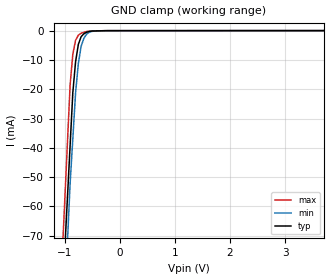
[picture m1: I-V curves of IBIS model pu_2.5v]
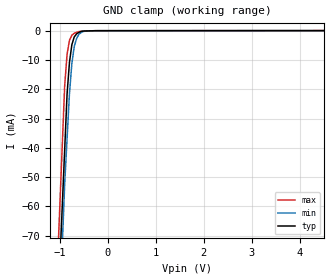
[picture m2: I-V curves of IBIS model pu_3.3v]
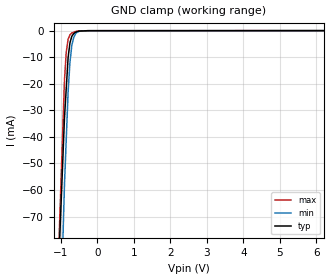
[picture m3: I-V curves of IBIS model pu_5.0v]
| Teraspeed Modeling Services.
| http://www.teraspeed.com
[IBIS Ver]   4.0
[Comment Char] |_char
[File Name]   pca9617dp.ibs
[File Rev]   3.0
[Source]  Measured and created by Teraspeed Consulting Group LLC
[Date]   10-19-2012
[Notes]   Quality Check of this IBIS model: Model Passes IBIS Check
   Model parses into ICX IS. Simulation done with Hyperlynx.
   1. MIN TYP MAX information is based on Temperature and Voltage
   characteristics only.
   2. Package data measured using Tektronix IConnect Software.
[Disclaimer]
| Use: Teraspeed Consulting Group LLC ("Teraspeed") has
| licensed IBIS models to specific integrated circuit
| suppliers ("IC Vendors") for use and distribution as
| follows: Each IC Vendor may use IBIS Models, and distribute
| them to IC Vendor's customers to use solely for developing
| printed circuit board designs. Users of this model may
| modify the IBIS model to suit its specific applications but
| rights to derivative works and such modifications shall belong
| to Teraspeed. No other distribution of these materials is
| permitted.
| DISCLAIMER OF WARRANTY: UNLESS OTHERWISE AGREED TO IN WRITING
| TERASPEED DISCLAIMS AND USER WAIVES ALL WARRANTIES, EXPRESS
| OR IMPLIED, INCLUDING WARRANTIES OF MERCHANTABILITY AND
| FITNESS FOR A PARTICULAR PURPOSE. IN NO EVENT SHALL
| TERASPEED BE LIABLE FOR ANY DIRECT OR INDIRECT DAMAGES,
| WHETHER IN CONTRACT OR TORT, INCLUDING, WITHOUT LIMITATION,
| LOST PROFITS, BUSINESS INTERRUPTION, OR LOST INFORMATION
| ARISING OUT OF THE USE OF OR THE INABILITY TO USE THE MODEL,
| EVEN IF TERASPEED HAS BEEN ADVISED OF THE POSSIBILITY OF SUCH
| DAMAGES.
[Copyright]
| This file is the legal property of Teraspeed Copyright(c) 2012.
| All other rights are reserved.
[Component] PCA9617DP
[Manufacturer] NXP Semiconductors
| TSSOP08/SOT505-1
[Package]
| variable   typ   min   max
R_pkg  1.100E-02  1.000E-02  1.200E-01
L_pkg  2.140E-09  2.040E-09  2.240E-09
C_pkg  5.910E-13  5.470E-13  6.350E-13
[Pin] signal_name  model_name  R_pin  L_pin C_pin
1  VCCA  POWER   1.200E-02 2.240E-09 5.470E-13
2  SCLA  io_side_a 1.000E-02 2.040E-09 6.350E-13
3  SDAA  io_side_a 1.000E-02 2.040E-09 6.350E-13
4  GND   GND   1.200E-02 2.240E-09 5.470E-13
5  EN   in_pu   1.200E-02 2.240E-09 5.470E-13
6  SDAB  io_side_b 1.000E-02 2.040E-09 6.350E-13
7  SCLB  io_side_b 1.000E-02 2.040E-09 6.350E-13
8  VCCB  POWER   1.200E-02 2.240E-09 5.470E-13
[Model selector] in_pu
pu_2.5v   input pin w/int pu,vccb=2.5v
pu_3.3v   input pin w/int pu,vccb=3.3v
pu_5.0v   input pin w/int pu,vccb=5.0v
[Model selector] io_side_b
sdab_2.5v  open drain io,vccb=2.5v
sdab_3.3v  open drain io,vccb=3.3v
sdab_5.0v  open drain io,vccb=5.0v
[Model selector] io_side_a
scla_0.95v  open drain io,vcca=0.95v
scla_1.8v   open drain io,vcca=1.8v
scla_2.5v   open drain io,vcca=2.5v
scla_3.3v   open drain io,vcca=3.3v
scla_5.0v   open drain io,vcca=5.0v
| Models and submodels in the file (11): pu_2.5v (Input), pu_3.3v (Input), pu_5.0v (Input), scla_0.95v (Open_drain), scla_1.8v (Open_drain), scla_2.5v (Open_drain), scla_3.3v (Open_drain), scla_5.0v (Open_drain), sdab_2.5v (Open_drain), sdab_3.3v (Open_drain), sdab_5.0v (Open_drain)
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[Model] pu_2.5v
Model_type Input
Vinl = 750.000mV
Vinh = 1.75000V
C_comp 600.000fF 595.000fF 605.000fF
| variable typ   min   max
[Voltage Range] 2.50000V 2.25000V 2.75000V
[POWER Clamp Reference] 2.50000V 2.25000V 2.75000V
[GND Clamp Reference] 0.00000V 0.00000V 0.00000V
[Temperature Range]   25   85   -40
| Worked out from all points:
|   GND clamp passes 1 mA (typ) near -0.64 V on its own axis
[GND Clamp]
-2.5V     -627.1mA   -717.8mA   -670.4mA
-900mV    -39.48mA   -52.45mA   -18.76mA
-850mV    -21.11mA   -36.83mA   -7.99mA
-800mV    -10.6mA    -21.21mA   -3.277mA
-750mV    -4.707mA   -11.24mA   -1.562mA
-700mV    -2.099mA   -5.37mA    -892uA
-650mV    -1.081mA   -2.621mA   -599.1uA
-600mV    -559.7uA   -1.191mA   -306.3uA
-550mV    -288.3uA   -553.5uA   -144.6uA
-450mV    -112.8uA   -112.5uA   -100.7uA
5V        11.01uA    12.15uA    11.05uA
[POWER Clamp]
-2.5V     0A         0A         0A
5V        0A         0A         0A
[Model] pu_3.3v
Model_type Input
Vinl = 990.000mV
Vinh = 2.31000V
C_comp 600.000fF 595.000fF 605.000fF
| variable typ   min   max
[Voltage Range] 3.30000V 2.97000V 3.63000V
[POWER Clamp Reference] 3.30000V 2.97000V 3.63000V
[GND Clamp Reference] 0.00000V 0.00000V 0.00000V
[Temperature Range]   25   85   -40
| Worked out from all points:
|   GND clamp passes 1 mA (typ) near -0.64 V on its own axis
[GND Clamp]
-3.3V     -958.1mA   -1.054A    -992.5mA
-900mV    -40.76mA   -52.47mA   -18.88mA
-850mV    -21.65mA   -36.93mA   -8.066mA
-800mV    -10.81mA   -21.4mA    -3.309mA
-750mV    -4.779mA   -11.22mA   -1.574mA
-700mV    -2.121mA   -5.352mA   -898.2uA
-650mV    -1.09mA    -2.612mA   -604.4uA
-600mV    -564.5uA   -1.187mA   -310.5uA
-550mV    -291.8uA   -553.5uA   -148.8uA
-450mV    -115.7uA   -113.5uA   -104.6uA
6.6V      16.4uA     15.45uA    14uA
[POWER Clamp]
-3.3V     0A         0A         0A
6.6V      0A         0A         0A
[Model] pu_5.0v
Model_type Input
Vinl = 1.50000V
Vinh = 3.50000V
C_comp 600.000fF 595.000fF 605.000fF
| variable typ   min   max
[Voltage Range] 5.00000V 4.50000V 5.50000V
[POWER Clamp Reference] 5.00000V 4.50000V 5.50000V
[GND Clamp Reference] 0.00000V 0.00000V 0.00000V
[Temperature Range]   25   85   -40
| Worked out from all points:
|   GND clamp passes 1 mA (typ) near -0.64 V on its own axis
[GND Clamp]
-5V       -1.459A    -2.026A    -1.674A
-900mV    -32.74mA   -57.89mA   -18.48mA
-850mV    -21.38mA   -40.39mA   -7.863mA
-800mV    -10.01mA   -22.89mA   -3.237mA
-750mV    -4.6mA     -11.87mA   -1.553mA
-700mV    -2.151mA   -5.589mA   -892.8uA
-650mV    -1.158mA   -2.704mA   -602.4uA
-600mV    -624.7uA   -1.224mA   -312uA
-500mV    -158.3uA   -269.2uA   -129.6uA
-225mV    -21.73uA   -24.81uA   -26.09uA
10V       17.25uA    24.22uA    16.58uA
[POWER Clamp]
-5V       0A         0A         0A
10V       0A         0A         0A
